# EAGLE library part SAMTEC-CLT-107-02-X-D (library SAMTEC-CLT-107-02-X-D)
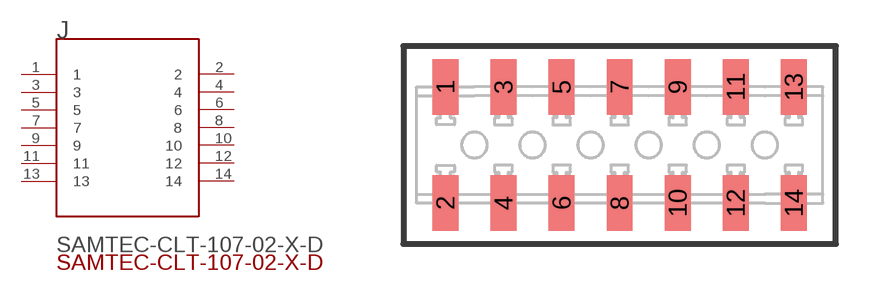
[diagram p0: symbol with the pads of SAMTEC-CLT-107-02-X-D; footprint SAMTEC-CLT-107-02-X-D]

Designator prefix J

## SAMTEC-CLT-107-02-X-DJ (Description: SOCKET, 2.0MM, SMT, 2X7POS; Series: -; Pitch Spacing: 2mm; No. of Rows: 2; No. of C; Digi-Key_Part_Number: SAM9249-ND; Digi-Key_Purchase_URL: https://www.digikey.com/product-detail/en/samtec-inc/CLT-107-02-L-D-BE/SAM9249-ND/6677986?utm_source=snapeda&utm_medium=aggregator&utm_campaign=symbol; MF: Samtec Inc.; MP: CLT-107-02-L-D; Package: None)  [SAMTEC-CLT-107-02-X-D]
1  1  pas
2  2  pas
3  3  pas
4  4  pas
5  5  pas
6  6  pas
7  7  pas
8  8  pas
9  9  pas
10  10  pas
11  11  pas
12  12  pas
13  13  pas
14  14  pas

## Footprint SAMTEC-CLT-107-02-X-D (pad centres in mm)
translated Allegro footprint
smd 0.89 x 1.91: 1 -6,2; 2 -6,-2; 3 -4,2; 4 -4,-2; 5 -2,2; 6 -2,-2; 7 0,2; 8 0,-2; 9 2,2; 10 2,-2; 11 4,2; 12 4,-2; 13 6,2; 14 6,-2

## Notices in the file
This work is licensed under a Creative Commons Attribution-ShareAlike 4.0 International License (CC BY-SA) with Design Exception 1.0
